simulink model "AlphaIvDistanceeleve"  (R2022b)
settings: Solver=FixedStepAuto  StartTime=0.0  StopTime=8/40000  FixedStep=1/40000000  RelTol=1e-3

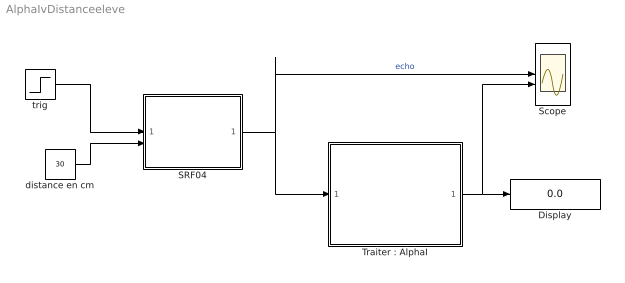
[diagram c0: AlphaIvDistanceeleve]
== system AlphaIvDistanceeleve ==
  Display : Display
  SRF04 : Subsystem
  Scope : Scope  NumInputPorts=2
  "Traiter : AlphaI" : Subsystem
  distance en cm : Constant  Value=30
  trig : Step  Time=6/400000  Before=1  After=0  SampleTime=0
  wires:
  trig/1 -> SRF04/1(Trig)
  SRF04/1(echo) -> "Traiter : AlphaI"/1(echo), Scope/1  "echo"
  distance en cm/1 -> SRF04/2(distance)
  "Traiter : AlphaI"/1(distance) -> Scope/2, Display/1

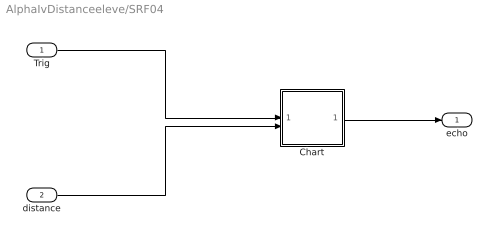
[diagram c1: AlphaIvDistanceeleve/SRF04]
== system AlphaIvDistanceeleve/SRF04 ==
  Trig : Inport
  distance : Inport  Port=2
  Chart : Stateflow chart  TreatAsAtomicUnit=on
  echo : Outport  VectorParamsAs1DForOutWhenUnconnected=off
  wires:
  Trig/1 -> Chart/1(trig)
  distance/1 -> Chart/2(d)
  Chart/1(echo) -> echo/1

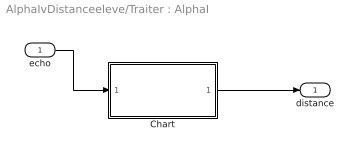
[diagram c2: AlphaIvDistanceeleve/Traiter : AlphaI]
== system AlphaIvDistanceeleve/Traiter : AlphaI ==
  echo : Inport
  Chart : Stateflow chart  TreatAsAtomicUnit=on
  distance : Outport
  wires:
  Chart/1(distance) -> distance/1
  echo/1 -> Chart/1(echo)

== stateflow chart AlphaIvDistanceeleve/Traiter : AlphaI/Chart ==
  state attente
    cpt=0;
  state affichage
  state comptage
    entry:
    cpt=cpt+1
    exit:
    distance=cpt/10
  (default) -> attente
  attente -> affichage : [echo]
  comptage -> affichage : [echo==1]
  affichage -> comptage : after(0.17,usec)
  comptage -> (junction 10) : [echo==0]
  data: echo input; distance output; cpt local

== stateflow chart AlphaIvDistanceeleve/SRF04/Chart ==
  state attente
    echo=0;
  state attente1
  state echo
    echo=1;
  (default) -> attente
  echo -> attente : after(0.0001*d/58,sec)
  attente -> attente1 : [trig==1]
  attente1 -> echo : after(0.0001,sec)
  data: trig input; d input; echo output
